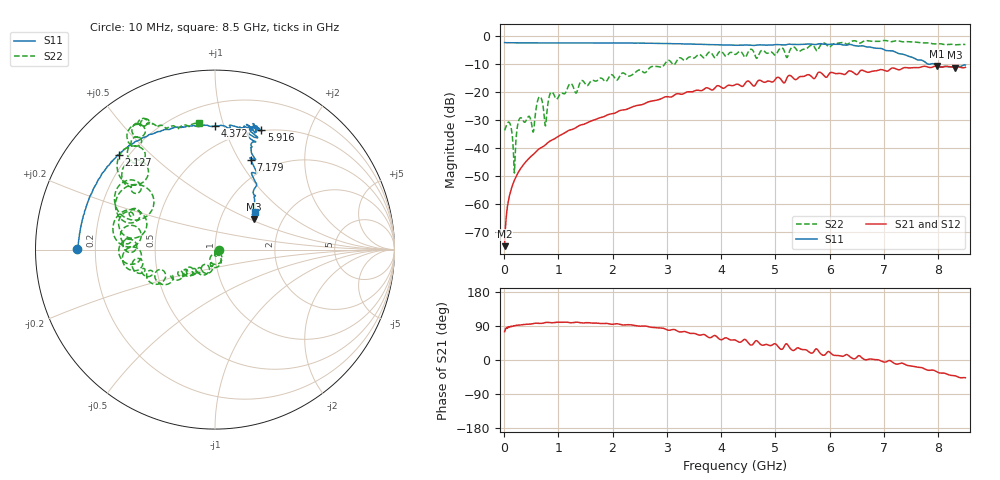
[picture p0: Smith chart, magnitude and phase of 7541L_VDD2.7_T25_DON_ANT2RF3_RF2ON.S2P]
!Agilent Technologies,E5071C,MY46417908,A.11.23
!Date: Wed Dec 09 17:17:42 2020
!Data & Calibration Information:
!Freq	S11:SOLT2(ON)	S21:SOLT2(ON)	S12:SOLT2(ON)	S22:SOLT2(ON)
!PortZ  Port1:50+j0  Port2:50+j0
!Above PortZ is port z conversion or system Z0 setting when saving the data.
!When reading, reference impedance value at option line is always used.
# Hz S dB R 50
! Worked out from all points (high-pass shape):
!   1601 points, 10 MHz to 8.5 GHz, reference 50 ohm
!   highest |S21| = -10.68 dB at 7.969 GHz (marker M1); lowest = -75.1 dB at 10 MHz (marker M2)
!   |S21| within 3 dB of the highest: 5.983 GHz to 6.255 GHz (271.8 MHz wide, 4.44 % of centre); 6.51 GHz to end of sweep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
!   lowest |S11| = -11.3 dB at 8.304 GHz (marker M3), VSWR 1.75, Z = 71.7 + j26.3 ohm
!   |S11| at or under -10 dB: 7.812058 GHz to 7.847164 GHz (35.11 MHz wide, 0.448 % of centre); 7.932 GHz to end of sweep
!   |S22| runs from -48.9 to -1.5 dB; largest |S21 - S12| = 0.0026
!   S11 on the Smith chart (normalised r, x): 10 MHz: 0.13, +0.00; 2.127 GHz: 0.16, +0.40; 4.372 GHz: 0.36, +0.93; 5.916 GHz: 0.49, +1.34; 7.179 GHz: 0.80, +1.12; 8.5 GHz: 1.39, +0.64
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1e7  -2.30 179.6  -75.11 74.8  -75.04 73.7  -33.71 0.1
1.002062e8  -2.35 177.6  -56.91 87.8  -57.00 87.7  -30.94 -53.3
1.904125e8  -2.37 175.3  -51.53 90.5  -51.57 90.4  -48.94 -39.1
3.177625e8  -2.40 172.5  -47.03 92.8  -47.00 92.7  -29.26 -60.9
5.300125e8  -2.41 167.7  -42.45 95.6  -42.43 95.8  -34.03 -78.4
6.520562e8  -2.42 165.3  -40.23 96.7  -40.23 96.7  -21.71 -80.9
7.634875e8  -2.43 162.6  -38.87 99.0  -38.88 99.1  -32.09 -85.2
8.696125e8  -2.42 160.1  -37.26 98.3  -37.25 98.5  -20.02 -87.5
1.426769e9  -2.41 148.6  -31.69 97.9  -31.69 97.8  -15.92 -118.4
2.127194e9  -2.46 135.4  -26.68 94.4  -26.67 94.4  -14.43 -132.6
2.843538e9  -2.59 123.0  -22.73 84.7  -22.74 84.7  -10.91 -150.2
4.255e9  -3.27 91.8  -17.40 52.9  -17.40 52.9  -6.52 174.1
4.371738e9  -3.22 90.0  -17.92 48.2  -17.93 48.1  -5.66 166.5
5.14645e9  -3.12 73.1  -16.65 31.8  -16.63 31.8  -4.63 142.0
5.247269e9  -2.87 75.4  -14.07 35.5  -14.06 35.5  -6.04 160.5
5.671769e9  -2.88 70.0  -14.61 18.2  -14.56 18.0  -3.24 135.9
5.915856e9  -2.93 68.8  -14.52 14.1  -14.48 14.1  -2.60 129.0
7.088538e9  -5.23 67.1  -12.25 -1.6  -12.30 -1.6  -1.88 118.0
7.178744e9  -5.41 68.1  -11.41 -7.9  -11.42 -7.7  -1.79 120.6
7.969375e9  -10.43 44.5  -10.68 -30.7  -10.70 -30.6  -2.76 111.8
8.303669e9  -11.25 38.3  -10.96 -41.4  -10.97 -41.3  -3.03 102.3
8.5e9  -10.34 43.4  -11.16 -46.7  -11.24 -46.6  -2.99 97.4
